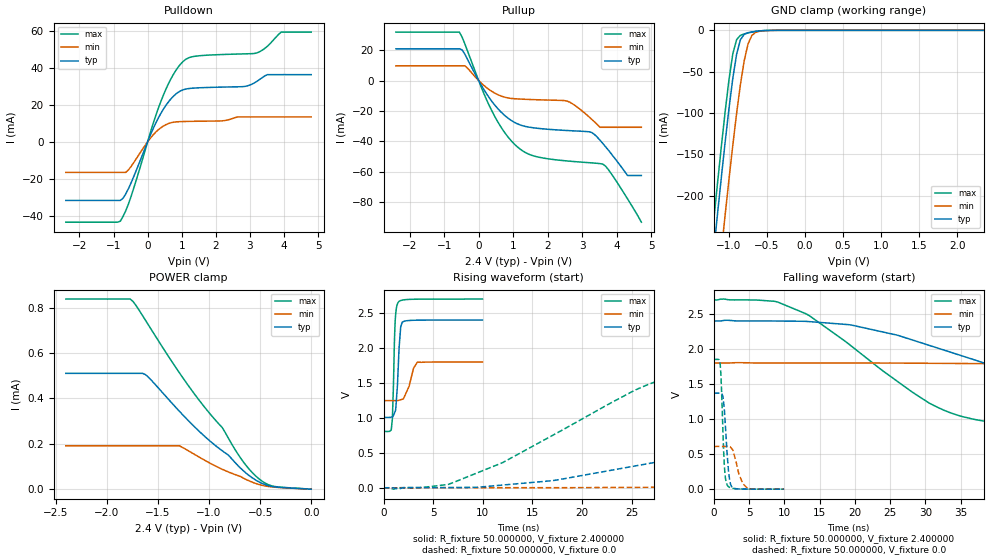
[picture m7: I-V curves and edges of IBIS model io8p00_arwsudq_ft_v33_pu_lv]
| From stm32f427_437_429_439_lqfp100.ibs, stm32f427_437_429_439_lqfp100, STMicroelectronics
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|   Model io8p00_arwsudq_ft_v33_pu_lv
[Model]  io8p00_arwsudq_ft_v33_pu_lv
Model_type I/O
Polarity   Non-Inverting
Enable   Active-Low
Vinl =   0.720000V
Vinh =   1.680000V
Vmeas =  1.200000V
Cref =   50.000000pF
Rref =   100.000000M
Vref =   0.0V
C_comp   2.828400pF   2.771400pF   2.910300pF
[Temperature Range]   25.000000   0.125000k   -40.000000
[Pullup Reference]   2.400000V   1.800000V   2.700000V
[Pulldown Reference]   0.0V   0.0V   0.0V
[POWER Clamp Reference]   2.400000V   1.800000V   2.700000V
[GND Clamp Reference]   0.0V   0.0V   0.0V
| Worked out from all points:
|   slope of the pulldown table from 0 to 0.36 V, typ, clamps not added: 25 ohm
|   slope of the pullup table from 0 to 0.36 V, typ, clamps not added: 27.7 ohm
|   GND clamp passes 1 mA (typ) near -0.62 V on its own axis
|   rising waveform, R_fixture 50.000000, V_fixture 2.400000: 20-80 % time 322ps typ, 710ps min, 219ps max; typ from 1.01 V to 2.4 V
|   rising waveform, R_fixture 50.000000, V_fixture 0.0: 20-80 % time 31ns typ, 81.8ns min, 14.6ns max; typ from 0.001 V to 1.37 V
|   falling waveform, R_fixture 50.000000, V_fixture 2.400000: 20-80 % time 29.1ns typ, 81.9ns min, 15.7ns max; typ from 2.4 V to 1.01 V
|   falling waveform, R_fixture 50.000000, V_fixture 0.0: 20-80 % time 552ps typ, 1.05ns min, 407ps max; typ from 1.37 V to 0.001 V
[Pulldown]
|Voltage   I(typ)   I(min)   I(max)
-2.4V     -31.66mA   -16.51mA   -43.42mA
-800mV    -31.66mA   -16.51mA   -42.86mA
-480mV    -21.98mA   -13.17mA   -29.21mA
80mV      3.63mA     1.966mA    5.014mA
480mV     18.16mA    8.738mA    26.02mA
800mV     25.38mA    10.72mA    37.77mA
1.12V     28.53mA    11.02mA    44.6mA
2.8V      29.84mA    13.46mA    47.53mA
3.2V      32.6mA     13.46mA    48.03mA
3.52V     36.33mA    13.46mA    51.75mA
3.92V     36.33mA    13.46mA    59.31mA
4.8V      36.33mA    13.46mA    59.31mA
[Pullup]
|Voltage   I(typ)   I(min)   I(max)
-2.4V     20.87mA    9.66mA     31.87mA
-560mV    20.87mA    9.66mA     31.87mA
-400mV    17.27mA    9.66mA     24.06mA
320mV     -11.75mA   -6.207mA   -17.08mA
640mV     -20.52mA   -10.1mA    -30.35mA
960mV     -26.47mA   -11.82mA   -40.02mA
1.52V     -30.88mA   -12.51mA   -49.05mA
2.56V     -32.88mA   -13.48mA   -52.9mA
3.28V     -34.2mA    -25.5mA    -54.17mA
3.6V      -41.33mA   -30.76mA   -54.99mA
4.32V     -62.5mA    -30.76mA   -77.87mA
4.72V     -62.5mA    -30.76mA   -93.2mA
[GND_clamp]
|Voltage   I(typ)   I(min)   I(max)
-2.4V     -1.428A    -1.51A     -1.401A
-1.2V     -266.4mA   -356.3mA   -229.4mA
-1.15V    -221.3mA   -311mA     -184.1mA
-1.1V     -177.3mA   -266.4mA   -140mA
-1.05V    -134.8mA   -222.7mA   -97.97mA
-950mV    -58.22mA   -139.2mA   -28.55mA
-900mV    -29.03mA   -100.6mA   -11.27mA
-850mV    -11.41mA   -65.77mA   -6.067mA
-750mV    -2.852mA   -16.63mA   -3.179mA
-700mV    -1.914mA   -6.318mA   -2.181mA
-600mV    -750uA     -1.167mA   -738.3uA
2.35V     0A         0A         0A
[POWER_clamp]
|Voltage   I(typ)   I(min)   I(max)
-2.4V     511uA      191.4uA    838.7uA
-1.77V    511uA      191.4uA    838.7uA
-1.74V    511uA      191.4uA    826.9uA
-1.62V    505.2uA    191.4uA    744.6uA
-1.29V    344.1uA    191.4uA    514uA
-1.08V    248.7uA    137.3uA    383.1uA
-870mV    169.3uA    87.75uA    271.7uA
-720mV    105.7uA    60.5uA     157.1uA
-570mV    47.98uA    29.54uA    70.06uA
-480mV    25.17uA    16.94uA    35.08uA
-390mV    12.49uA    10.17uA    15.15uA
0V        0A         0A         0A
[Ramp]
| variable   typ   min   max
dV/dt_r  0.82201/30.92306n   0.36326/83.85166n   1.11083/14.60523n
dV/dt_f  0.83748/29.14535n   0.32652/82.10536n   1.13677/15.69812n
R_load = 50.000000
[Rising Waveform]
R_fixture= 50.000000
V_fixture= 2.400000
V_fixture_min= 1.800000
V_fixture_max= 2.700000
|time   V(typ)   V(min)   V(max)
0s        1.007V     1.247V     805.7mV
780.8ps   1.013V     1.247V     845.7mV
880.9ps   1.017V     1.247V     988.5mV
1.161ns   1.093V     1.247V     2.383V
1.381ns   1.447V     1.247V     2.627V
1.481ns   1.758V     1.25V      2.656V
1.722ns   2.302V     1.26V      2.678V
1.882ns   2.371V     1.267V     2.685V
3.403ns   2.398V     1.797V     2.698V
9.97ns    2.4V       1.8V       2.7V
[Rising Waveform]
R_fixture= 50.000000
V_fixture= 0.0
V_fixture_min= 0.0
V_fixture_max= 0.0
|time   V(typ)   V(min)   V(max)
0s        880.4uV    840.2uV    911.2uV
7.007ns   4.465mV    1.891mV    74.99mV
17.02ns   102.3mV    2.04mV     748.6mV
28.03ns   380.4mV    8.553mV    1.547V
35.04ns   574.9mV    17.63mV    1.724V
43.04ns   805.9mV    44.83mV    1.794V
59.56ns   1.174V     100.9mV    1.84V
79.58ns   1.316V     194.9mV    1.848V
152.7ns   1.369V     510.6mV    1.852V
249.2ns   1.371V     610.3mV    1.852V
[Falling Waveform]
R_fixture= 50.000000
V_fixture= 2.400000
V_fixture_min= 1.800000
V_fixture_max= 2.700000
|time   V(typ)   V(min)   V(max)
0s        2.4V       1.8V       2.7V
9.009ns   2.399V     1.8V       2.672V
13.51ns   2.391V     1.8V       2.478V
19.52ns   2.342V     1.8V       2.041V
31.03ns   2.036V     1.796V     1.203V
43.54ns   1.625V     1.776V     913.9mV
60.56ns   1.236V     1.717V     846.3mV
84.08ns   1.083V     1.587V     819.3mV
157.7ns   1.014V     1.325V     806mV
249.2ns   1.007V     1.247V     805.7mV
[Falling Waveform]
R_fixture= 50.000000
V_fixture= 0.0
V_fixture_min= 0.0
V_fixture_max= 0.0
|time   V(typ)   V(min)   V(max)
0s        1.371V     610.3mV    1.852V
900.9ps   1.372V     610.1mV    1.792V
1.081ns   1.368V     610mV      1.463V
1.481ns   1.155V     609.7mV    368.9mV
1.922ns   470.1mV    610.9mV    56.85mV
2.262ns   120.9mV    607.9mV    25.02mV
2.743ns   18.52mV    545.4mV    12.12mV
3.584ns   3.983mV    209.2mV    5.051mV
4.785ns   1.869mV    11.65mV    2.214mV
9.97ns    880.4uV    840.2uV    911.2uV
